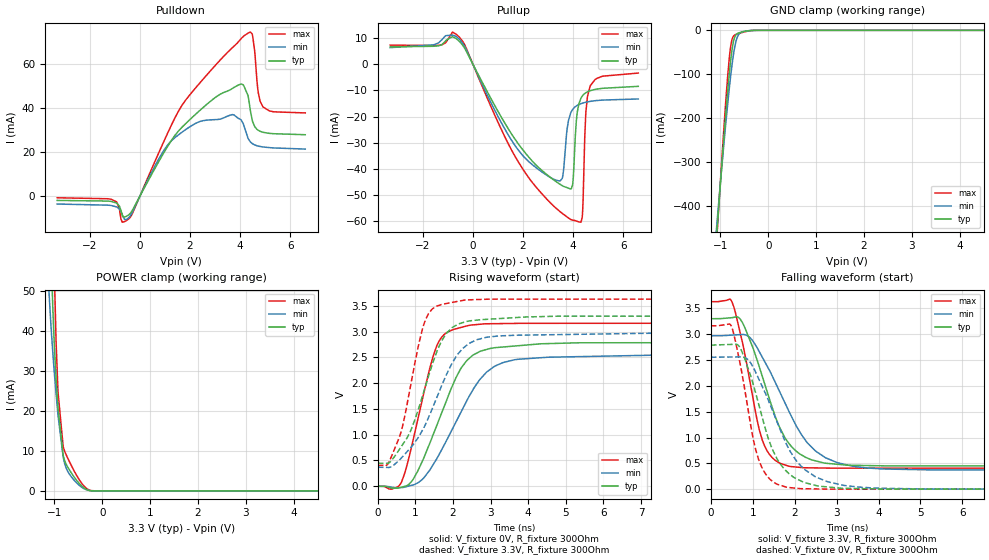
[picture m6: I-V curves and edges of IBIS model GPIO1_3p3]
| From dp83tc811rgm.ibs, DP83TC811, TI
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|   GPIO1_3p3 Model
[Model]   GPIO1_3p3
Model_type   I/O
Polarity   Non-Inverting
Enable   Active-Low
Vinl = 0.8
Vinh = 2
Vmeas = 1.65
Vref = 0
Cref = 2pF
Rref = 100000
|   typ   min   max
C_comp   6.9770pF   5.0542pF   9.1978pF
| Where Nom  PVT is Nominal Process, 3.3V, 27C
|   Fast PVT is Strong Process,  3.63V, -40C
|   Slow PVT is Weak Process,   2.97V, 125C
[Voltage Range]   3.3   2.97   3.63
|Junction Temperature
[Temperature Range]   27   125   -40
[Pullup Reference]   3.3   2.97   3.63
[Pulldown Reference]   0   0   0
[Power Clamp Reference]   3.3   2.97   3.63
[GND Clamp Reference]   0   0   0
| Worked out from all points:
|   slope of the pulldown table from 0 to 0.495 V, typ, clamps not added: 47.3 ohm
|   slope of the pullup table from 0 to 0.495 V, typ, clamps not added: 54.4 ohm
|   GND clamp passes 1 mA (typ) near -0.41 V on its own axis
|   POWER clamp passes 1 mA (typ) near -0.41 V on its own axis
|   falling waveform, V_fixture 3.3V, R_fixture 300Ohm: 20-80 % time 745ps typ, 1.01ns min, 479ps max; typ from 3.3 V to 0.449 V
|   rising waveform, V_fixture 0V, R_fixture 300Ohm: 20-80 % time 942ps typ, 1.14ns min, 621ps max; typ from 0 V to 2.79 V
|   rising waveform, V_fixture 3.3V, R_fixture 300Ohm: 20-80 % time 806ps typ, 1.01ns min, 548ps max; typ from 0.449 V to 3.3 V
|   falling waveform, V_fixture 0V, R_fixture 300Ohm: 20-80 % time 667ps typ, 886ps min, 446ps max; typ from 2.79 V to 0 V
[Pulldown]
|   Voltage   I(typ)   I(min)   I(max)
-3.3V     -1.922mA   -3.573mA   -721.5uA
-1.152V   -2.369mA   -4.234mA   -1.367mA
-706.2mV  -8.541mA   -8.263mA   -11.8mA
-429mV    -8.362mA   -9.653mA   -10.16mA
1.016V    20.95mA    21.88mA    26.44mA
2.095V    35.97mA    32.35mA    47.59mA
4.046V    51.14mA    34.69mA    71.86mA
4.412V    38.85mA    24.72mA    74.76mA
4.58V     31.77mA    23.36mA    66.24mA
4.729V    29.99mA    22.81mA    46.87mA
4.907V    29.14mA    22.44mA    40.78mA
6.6V      28.01mA    21.47mA    37.94mA
[GND Clamp]
|   Voltage   I(typ)   I(min)   I(max)
-3.3V     -4.085A    -3.538A    -4.624A
-1.073V   -458mA     -438.5mA   -468.1mA
-1.043V   -413.1mA   -400.7mA   -416.3mA
-884.4mV  -185.5mA   -208mA     -155.3mA
-844.8mV  -134.5mA   -163.9mA   -99.33mA
-795.3mV  -78.13mA   -112.8mA   -44.06mA
-755.7mV  -42.9mA    -76.82mA   -19.91mA
-716.1mV  -20.54mA   -47.14mA   -11.72mA
-676.5mV  -10.47mA   -25.72mA   -9.163mA
-627mV    -6.274mA   -11.03mA   -7.365mA
-260.7mV  -48.6uA    -53.84uA   -61.26uA
6.6V      0A         0A         0A
[Pullup]
|   Voltage   I(typ)   I(min)   I(max)
-3.3V     6.638mA    6.338mA    7.299mA
-537.9mV  8.729mA    9.539mA    10.32mA
1.541V    -26.61mA   -29mA      -32.74mA
2.927V    -41.93mA   -42.23mA   -51.26mA
3.561V    -46.31mA   -43.65mA   -56.87mA
3.897V    -47.58mA   -18.74mA   -59.18mA
4.155V    -19.08mA   -15.75mA   -59.91mA
4.313V    -12.91mA   -15.05mA   -60.27mA
4.382V    -11.91mA   -14.83mA   -55.35mA
4.511V    -10.84mA   -14.5mA    -17.94mA
4.679V    -10.09mA   -14.17mA   -8.311mA
6.6V      -8.433mA   -13.25mA   -3.368mA
[POWER Clamp]
|   Voltage   I(typ)   I(min)   I(max)
-3.3V     2.109A     1.785A     2.366A
-1.112V   82.02mA    49.75mA    135mA
-1.063V   57.26mA    39.83mA    95.49mA
-1.033V   45.98mA    34.71mA    74.36mA
-1.003V   37.11mA    29.99mA    56.06mA
-963.6mV  27.98mA    24.2mA     37.24mA
-924mV    20.83mA    18.95mA    24.8mA
-815.1mV  8.873mA    8.438mA    10.98mA
-755.7mV  6.746mA    5.802mA    9.104mA
-676.5mV  5.087mA    4.045mA    7.098mA
-339.9mV  432.5uA    346.3uA    736.8uA
6.6V      0A         0A         0A
[Ramp]
R_load = 300
|   typ   min   max
dV/dt_r   1.67347/9.38904e-10   1.5336/1.13581e-09   1.89785/6.21098e-10
dV/dt_f   1.71076/7.45393e-10   1.55992/1.01093e-09   1.93409/4.75128e-10
[Falling Waveform]
V_fixture = 3.3V
V_fixture_min = 2.97V
V_fixture_max = 3.63V
R_fixture = 300Ohm
C_fixture = 0F
|   Time   V(typ)   V(min)   V(max)
0s        3.3V       2.97V      3.63V
474.6ps   3.318V     2.981V     3.667V
754.2ps   3.224V     2.995V     2.838V
1.095ns   2.52V      2.752V     1.373V
1.231ns   2.175V     2.55V      944mV
1.473ns   1.56V      2.177V     602mV
1.857ns   890.7mV    1.517V     444.7mV
2.496ns   548.8mV    738.8mV    411.5mV
3.71ns    457.7mV    411.3mV    406.7mV
20ns      448.6mV    370mV      406.3mV
[Rising Waveform]
V_fixture = 0V
V_fixture_min = 0V
V_fixture_max = 0V
R_fixture = 300Ohm
C_fixture = 0F
|   Time   V(typ)   V(min)   V(max)
0s        25.41uV    64.36uV    17.49uV
573.3ps   -28.07mV   -28.54mV   15.96mV
928.5ps   124.4mV    23.73mV    866.2mV
1.371ns   814mV      302.3mV    2.256V
1.591ns   1.223V     564.1mV    2.761V
2.077ns   2.105V     1.246V     3.053V
2.373ns   2.443V     1.668V     3.111V
3.124ns   2.688V     2.334V     3.153V
4.514ns   2.766V     2.502V     3.16V
20ns      2.789V     2.556V     3.163V
[Rising Waveform]
V_fixture = 3.3V
V_fixture_min = 2.97V
V_fixture_max = 3.63V
R_fixture = 300Ohm
C_fixture = 0F
|   Time   V(typ)   V(min)   V(max)
0s        448.6mV    370mV      406.3mV
298.3ps   456.8mV    364.7mV    473.6mV
603.9ps   748.3mV    530.7mV    1.019V
782.4ps   944.1mV    674.6mV    1.606V
1.227ns   1.846V     1.14V      3.146V
1.447ns   2.359V     1.502V     3.437V
1.721ns   2.847V     1.991V     3.53V
2.254ns   3.172V     2.67V      3.603V
3.219ns   3.251V     2.915V     3.628V
20ns      3.3V       2.97V      3.63V
[Falling Waveform]
|Gnd
V_fixture = 0V
V_fixture_min = 0V
V_fixture_max = 0V
R_fixture = 300Ohm
C_fixture = 0F
|   Time   V(typ)   V(min)   V(max)
0s        2.789V     2.554V     3.163V
466ps     2.802V     2.558V     3.187V
680.1ps   2.761V     2.56V      2.498V
1.01ns    2.03V      2.359V     972.7mV
1.153ns   1.61V      2.116V     545.8mV
1.459ns   786.7mV    1.545V     158.2mV
1.798ns   351.8mV    879.5mV    38.92mV
2.508ns   70.92mV    234.3mV    4.795mV
3.933ns   5.258mV    20.45mV    563.9uV
20ns      25.36uV    63.89uV    17.64uV
